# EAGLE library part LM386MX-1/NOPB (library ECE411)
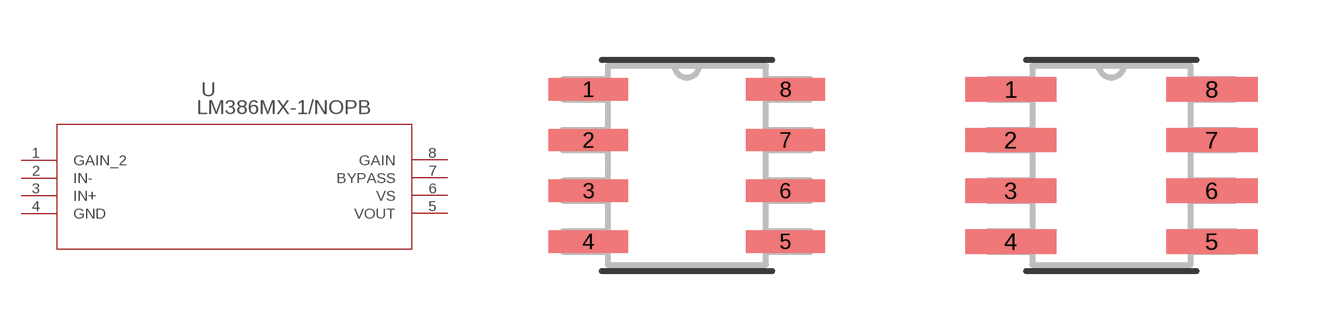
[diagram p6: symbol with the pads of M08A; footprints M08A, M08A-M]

Designator prefix U

## LM386MX-1/NOPB (MANUFACTURER_PART_NUMBER: LM386MX1NOPB; VENDOR: Texas Instruments)  [M08A]
1  GAIN_2  pas
2  IN-  in
3  IN+  in
4  GND  pwr
5  VOUT  out
6  VS  pwr
7  BYPASS  pas
8  GAIN  pas

## LM386MX-1/NOPBM08A-M (MANUFACTURER_PART_NUMBER: LM386MX1NOPB; VENDOR: Texas Instruments)  [M08A-M]
Pads as for M08A

## LM386MX-1/NOPBM08A-L (MANUFACTURER_PART_NUMBER: LM386MX1NOPB; VENDOR: Texas Instruments)  [M08A-L]
Pads as for M08A

## Footprint M08A (pad centres in mm)
smd 1.981 x 0.559: 1 -2.464,1.905; 2 -2.464,0.635; 3 -2.464,-0.635; 4 -2.464,-1.905; 5 2.464,-1.905; 6 2.464,-0.635; 7 2.464,0.635; 8 2.464,1.905

## Footprint M08A-M (pad centres in mm)
smd 2.286 x 0.61: 1 -2.515,1.905; 2 -2.515,0.635; 3 -2.515,-0.635; 4 -2.515,-1.905; 5 2.515,-1.905; 6 2.515,-0.635; 7 2.515,0.635; 8 2.515,1.905

## Footprint M08A-L (pad centres in mm)
smd 1.676 x 0.508: 1 -2.413,1.905; 2 -2.413,0.635; 3 -2.413,-0.635; 4 -2.413,-1.905; 5 2.413,-1.905; 6 2.413,-0.635; 7 2.413,0.635; 8 2.413,1.905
